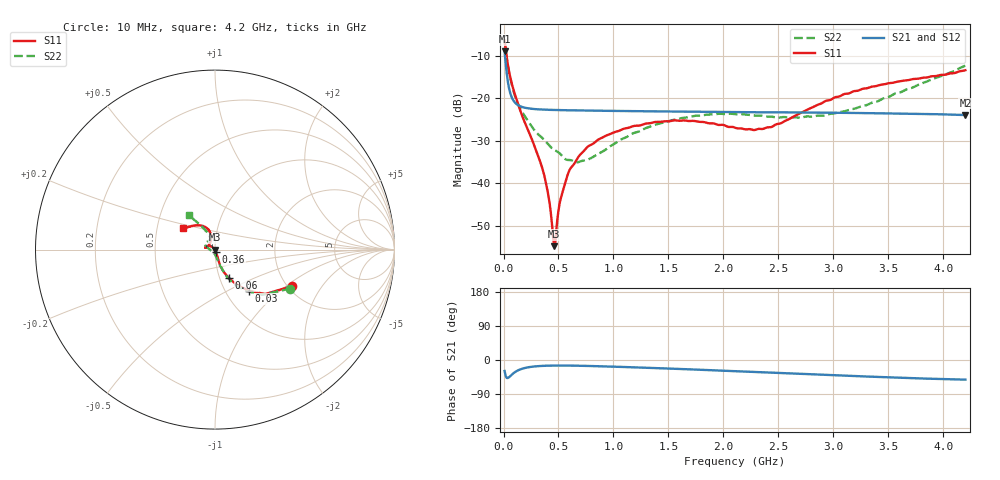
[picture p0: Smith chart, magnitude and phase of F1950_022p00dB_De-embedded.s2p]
! Integrated Device Technology
! Corporate Headquarters
! 6024 Silver Creek Valley Road
! San Jose, CA 95138  USA
! Phone:  1-408-284-8200
! Toll Free:  1-800-223-1366
! Webpage:  http://www.idt.com/
! Timing and RF Division
! 515 Groton Road, Suite 102
! Westford, MA 01886-6024
! Device:  F1950
! Description: 7-bit 0.25 dB Digital Step Attenuator
! Frequency:  150.0 -  4000.00 MHz
! Package:  4x4 mm Thin QFN Plastic Package: 24 pin
! Ports:  2 RF, 12 DC
!  Pin  1  = D0
!  Pin  2  = VDD
!  Pin  3  = Vmode
!  Pin  4  = GND
!  Pin  5  = RF1  =  Port 1
!  Pin  6  = GND
!  Pin  7  = GND
!  Pin  8  = GND
!  Pin  9  = GND
!  Pin 10  = GND
!  Pin 11  = GND
!  Pin 12  = GND
!  Pin 13  = GND
!  Pin 14  = RF2  =  Port 2
!  Pin 15  = GND
!  Pin 16  = LE
!  Pin 17  = CLK
!  Pin 18  = DATE
!  Pin 19  = D6
!  Pin 20  = D5
!  Pin 21  = D4
!  Pin 22  = D3
!  Pin 23  = D2
!  Pin 24  = D1
! State:  88
! Atten State:  22.00 dB
! Voltage:  +5.00 Volts
! Current:  Not Measured mA
! Data:  The device was measured on a the F195X evaluation board which has
!  individual transmission lines to the RF pins.  Data was collected
!  using a calibrated network analyzer.  The evaluation board was
!  de-embedded using a TRL calibration technique.
!  The reference plane is the edge of the package pin.
! Misc:  Board 2019
!  Action Tracker AT0250
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# GHz S dB R 50
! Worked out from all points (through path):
!   420 points, 10 MHz to 4.2 GHz, reference 50 ohm
!   highest |S21| = -9.05 dB at 10 MHz (marker M1); lowest = -24.0 dB at 4.2 GHz (marker M2)
!   group delay of S21, straight-line fit = 24.7 ps
!   lowest |S11| = -54.8 dB at 460 MHz (marker M3), VSWR 1.00, Z = 49.9 - j0.115 ohm
!   |S11| at or under -10 dB: 27.52 MHz to end of sweep
!   |S22| runs from -35.1 to -6.5 dB; largest |S21 - S12| = 0.00013
!   S11 on the Smith chart (normalised r, x): 10 MHz: 2.11, -1.11; 30 MHz: 1.29, -0.65; 60 MHz: 1.11, -0.37; 360 MHz: 1.01, -0.03; 4.2 GHz: 0.68, +0.17
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0.01  -6.46 -25.3  -9.05 -28.9  -9.04 -28.9  -6.51 -27.4
0.03  -10.48 -50.4  -14.31 -47.4  -14.31 -47.4  -10.75 -52.7
0.06  -14.95 -63.6  -18.72 -42.9  -18.72 -42.9  -15.09 -65.1
0.1  -18.82 -70.3  -20.92 -32.8  -20.92 -32.8  -19.15 -70.3
0.15  -22.77 -72.3  -21.89 -25.0  -21.89 -25.0  -22.37 -74.5
0.36  -37.16 -70.2  -22.70 -15.4  -22.70 -15.4  -29.56 -85.4
0.4  -41.73 -75.0  -22.74 -15.0  -22.74 -15.0  -30.65 -87.1
0.45  -52.43 -109.6  -22.78 -14.7  -22.78 -14.7  -31.96 -93.4
0.46  -54.78 -141.0  -22.79 -14.7  -22.79 -14.7  -32.14 -95.1
0.48  -51.06 159.9  -22.80 -14.6  -22.80 -14.6  -32.43 -98.0
0.52  -43.64 142.9  -22.82 -14.6  -22.82 -14.6  -33.21 -101.6
0.58  -38.27 136.5  -22.85 -14.7  -22.85 -14.7  -34.52 -114.0
0.71  -32.95 138.7  -22.90 -15.3  -22.90 -15.3  -34.77 -139.1
0.99  -28.21 148.0  -23.01 -17.5  -23.00 -17.6  -31.00 -179.0
1.41  -25.59 163.6  -23.12 -21.7  -23.12 -21.7  -26.02 161.6
1.73  -25.35 169.1  -23.19 -25.1  -23.18 -25.1  -24.22 153.2
2.11  -27.00 159.1  -23.27 -29.6  -23.27 -29.6  -23.78 143.6
2.43  -26.83 127.6  -23.33 -33.1  -23.33 -33.1  -24.35 133.2
2.81  -22.17 106.1  -23.40 -37.8  -23.40 -37.8  -24.35 117.9
3.1  -19.03 107.6  -23.46 -41.2  -23.46 -41.3  -23.11 112.8
3.51  -16.48 118.0  -23.58 -45.8  -23.57 -45.9  -19.64 114.3
4.2  -13.45 146.1  -23.98 -51.7  -23.97 -51.8  -12.38 127.5
